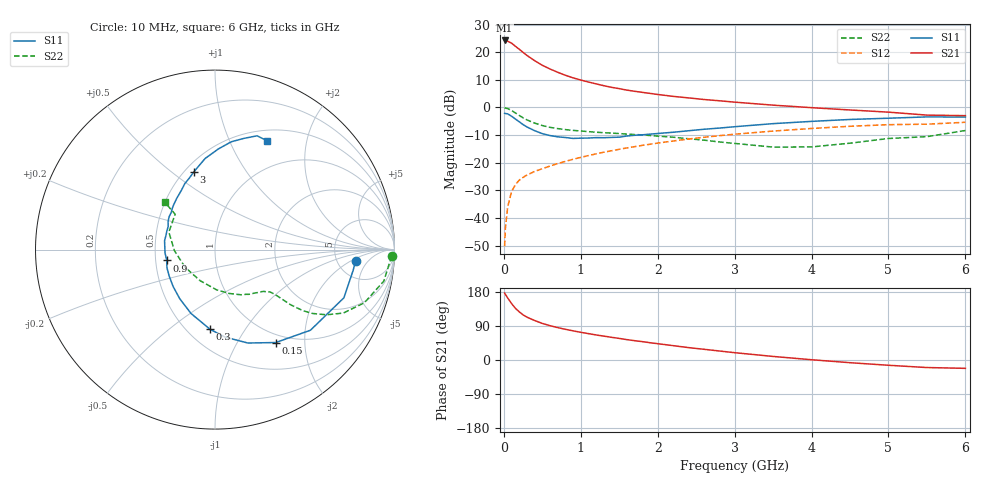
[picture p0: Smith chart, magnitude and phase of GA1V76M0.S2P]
! Infineon Technologies  Discrete & RF Semiconductors
! BF775
! Si NPN RF Bipolar Junction Transistor in SOT23
! VCE = 1.75 V  IC = 6 mA
! Common Emitter S-Parameters:  May  1996
# GHz  S  MA  R  50
!  f  S11  S21  S12  S22
! GHz  MAG  ANG  MAG  ANG  MAG  ANG  MAG  ANG
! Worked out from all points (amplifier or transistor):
!   36 points, 10 MHz to 6 GHz, reference 50 ohm
!   highest |S21| = 24.3 dB at 10 MHz (marker M1)
!   |S21| within 3 dB of that: start of sweep to 192.2 MHz
!   unconditionally stable (mu >= 1): 689.2 MHz to 4.062 GHz; 5.275 GHz to 5.874 GHz
!   at 250 MHz: K = 0.55, MSG = 22.6 dB, |S12| = -25.3 dB
!   at 1.4 GHz: K = 1.15, MAG = 9.1 dB, |S12| = -15.7 dB
!   at 6 GHz: K = 1.00, MSG = 1.2 dB, |S12| = -5.3 dB
!   S11 on the Smith chart (normalised r, x): 10 MHz: 7.55, -2.44; 150 MHz: 0.88, -1.47; 300 MHz: 0.64, -0.71; 900 MHz: 0.57, -0.08; 3 GHz: 0.56, +0.60; 6 GHz: 0.63, +1.39
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0.01  0.7862 -4.5  16.32 176.8  0.0031 90.4  0.987 -2.1
0.02  0.7784 -8.5  16.15 173.2  0.0065 85.4  0.9754 -4.3
0.05  0.7667 -20.5  15.8 163.7  0.0159 79.4  0.9566 -10.6
0.1  0.6961 -40.2  14.61 149.1  0.03 70.7  0.8834 -19.6
0.15  0.6187 -56.8  12.81 136.6  0.0403 64.0  0.7977 -26.3
0.2  0.5519 -70.6  11.34 127.1  0.0484 60.4  0.7199 -30.3
0.25  0.4908 -83.4  9.931 119.1  0.0544 57.5  0.6497 -33.2
0.3  0.445 -93.5  8.755 113.1  0.06 56.3  0.5963 -34.8
0.4  0.3804 -110.5  7.039 104.2  0.0698 55.3  0.5226 -36.1
0.5  0.3368 -125.7  5.808 96.5  0.0781 55.4  0.4719 -36.4
0.6  0.3107 -138.8  4.974 90.6  0.0872 56.2  0.4376 -36.6
0.7  0.295 -149.8  4.338 85.5  0.0966 56.7  0.4155 -36.9
0.9  0.2757 -167.3  3.437 76.9  0.1158 57.1  0.3855 -37.7
1.1  0.2801 177.0  2.889 69.6  0.1351 57.3  0.3659 -39.8
1.3  0.2843 164.5  2.479 63.0  0.1555 56.7  0.3501 -42.0
1.6  0.3049 149.0  2.062 53.7  0.1855 55.1  0.33 -46.9
2.2  0.3566 126.7  1.59 37.9  0.2477 50.1  0.2904 -60.1
3  0.4491 105.2  1.25 19.3  0.3288 40.9  0.224 -87.9
3.5  0.5105 96.2  1.103 9.4  0.3745 34.5  0.192 -115.4
4.5  0.6076 81.4  0.902 -7.1  0.4573 21.1  0.2262 -178.6
5.5  0.676 69.7  0.728 -19.9  0.4991 6.7  0.2969 138.4
6  0.6723 64.6  0.712 -22.0  0.5404 2.7  0.3833 136.7
